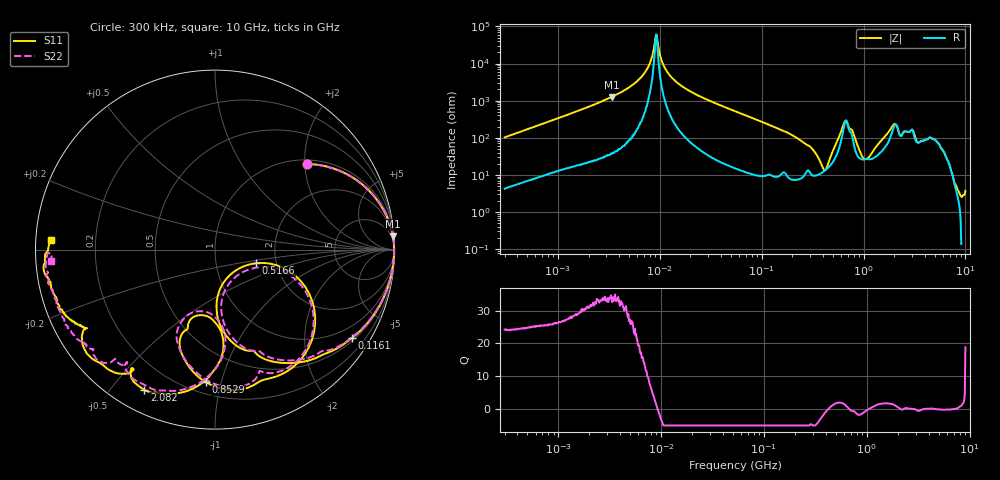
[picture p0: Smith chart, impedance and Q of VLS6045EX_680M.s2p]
! S-Parameter Data Generated by TDK Corporation
! Copyright(C) 2019 TDK Corporation.
! All Rights Reserved.
! TDK P/N: VLS6045EX-680M (Inductor)
! Property: L=68uH at 100kHz
! Size(LxWxT): 6x6x4.5mm
! Model Type: s2p (Touchstone File Format Version 1.0)
! Frequency: DC=Yes Start=0.3MHz Stop=10000MHz 802points Log-sweep
! Model Generated on May 10, 2019
! Port Assignments:
!  1 ---@@@--- 2
! Applicable Conditions:
!  Temperature = 25 degC
!  DC Bias Current = 0 A
!  Small Signal Operation
! Terms and conditions regarding TDK Simulation Models
! (1)This simulation model is being provided solely for informational purposes. Please refer to the specifications of the products in terms of detailed characteristics of such products.
! (2)In no event shall TDK Corporation of any of its subsidiaries be liable for any loss or damage arising, directly or indirectly,
!  From any information contained in this simulation model, including, but not limited to loss or damages arising from any inaccuracies, omissions or errors in connection with such information.
! (3)Any and all copyrights on this simulation model are owned by TDK Corporation.
!  Duplication or redistribution of this simulation model without prior written permission from TDK Corporation is prohibited.
! (4)This simulation model is subject to any modification or change without any prior notice.
! (5)Neither TDK Corporation nor any of its subsidiaries shall make any warranty, express or implied,
!  Including but not limited to the correctness, implied warranties of merchantability and fitness for a particular purpose with respect to this simulation models.
! (6)The use of this simulation model shall be deemed to have consented to the terms and conditions hereof.
# Hz S MA R 50
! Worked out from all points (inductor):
!   801 points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, 300 kHz to 10 GHz, reference 50 ohm
!   read as one part in series: L = 53.9 uH near 318.3 kHz
!   highest Q = 33.7 at 3.375 MHz (marker M1), where L = 59.3 uH
!   self-resonance near 9.197 MHz
!   S11 on the Smith chart (normalised r, x): 300 kHz: 1.09, +2.05; 116.1 MHz: 0.59, -3.32; 516.6 MHz: 1.57, -0.25; 852.9 MHz: 0.27, -0.90; 2.082 GHz: 0.09, -0.61; 10 GHz: 0.04, +0.03
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300000  0.6998 43.1  0.686 -44.6  0.6861 -44.6  0.6994 43.0
1713600  0.9799 9.6  0.1694 -78.5  0.1695 -78.5  0.98 9.6
3374880  0.9944 4.2  0.07908 -84.0  0.07912 -84.1  0.9946 4.3
6556275  0.9981 0.7  0.02336 -85.6  0.02335 -85.6  0.9983 0.8
8009306  0.9983 -0.2  0.009679 -80.9  0.009675 -80.9  0.9985 -0.1
9078145  0.9984 -0.7  0.001948 -38.2  0.001952 -37.9  0.9985 -0.7
9671944  0.9982 -1.1  0.003472 60.8  0.003476 60.9  0.9985 -1.0
1.092564e7  0.9981 -1.6  0.01133 79.8  0.01133 79.7  0.9984 -1.6
1.470778e7  0.9974 -3.2  0.03196 83.4  0.03195 83.3  0.9976 -3.1
5.477226e7  0.9772 -15.6  0.1857 73.0  0.1857 73.0  0.9774 -15.2
1.161426e8  0.9084 -32.6  0.3799 55.3  0.3799 55.3  0.9096 -31.9
3.126428e8  0.5692 -75.3  0.746 8.2  0.7459 8.1  0.5751 -72.9
4.687561e8  0.1691 -64.8  0.8277 -33.4  0.8276 -33.4  0.1945 -60.2
5.165633e8  0.2418 -18.3  0.7616 -49.4  0.7616 -49.4  0.2664 -21.6
6.325141e8  0.7189 -39.9  0.3063 -75.0  0.3063 -75.0  0.7218 -41.7
8.528959e8  0.7413 -93.8  0.4516 -19.5  0.4517 -19.5  0.7499 -89.9
1.038183e9  0.5013 -111.3  0.5867 -45.8  0.587 -45.8  0.5724 -110.9
1.276148e9  0.3719 -100.6  0.6144 -78.9  0.6146 -78.9  0.3512 -102.1
1.767019e9  0.7718 -97.8  0.2456 -139.1  0.246 -139.0  0.7762 -99.8
2.08171e9  0.8753 -116.7  0.1005 -113.8  0.1012 -113.9  0.8523 -121.0
3.219363e9  0.9074 -144.4  0.09535 -94.7  0.09491 -94.9  0.8947 -139.3
1e10  0.9171 176.6  0.05862 -159.7  0.05855 -159.7  0.9136 -176.1
